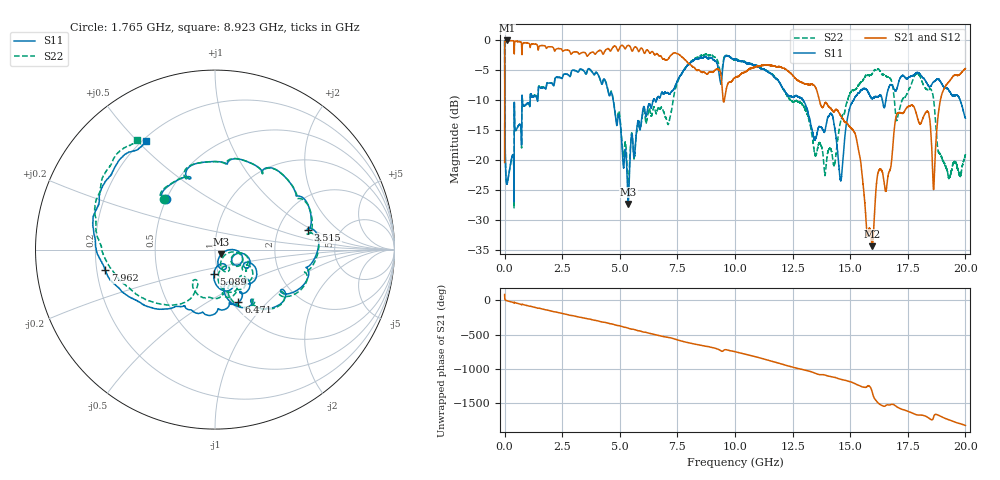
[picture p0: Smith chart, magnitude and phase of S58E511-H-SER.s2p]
!{S58E511}
!Johanson Technology Inc.
!www.johansontechnology.com
!Test Board Conditions:
!Substrate Type  RO4350B
!Substrate Thickness  60 mil
!Substrate Dk  3.66
!TL Type: GCPW
!TL Trace Width  115 mil
!TL Gap  52 mil
!Electrode orientation  Horizontal
!DUT TOPOLOGY	SERIES
!Mounting Pad LxW  55x428 mil
! Created Wed Apr 14 11:55:38 2021
# mhz S ma R 50
! 2 Port Network Data from SP1.SP block
! freq  magS11  angS11  magS21  angS21  magS12  angS12  magS22  angS22
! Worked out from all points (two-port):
!   20001 points, 300 kHz to 20 GHz, reference 50 ohm
!   highest |S21| = -0.02 dB at 99.3 MHz (marker M1); lowest = -34.4 dB at 15.95 GHz (marker M2)
!   |S21| within 3 dB of the highest: 3.17 MHz to 6.845 GHz (6.841 GHz wide, 200 % of centre); 7.119 GHz to 7.771 GHz (651.1 MHz wide, 8.75 % of centre)
!   lowest |S11| = -27.4 dB at 5.367 GHz (marker M3), VSWR 1.09, Z = 53.4 - j2.86 ohm
!   |S11| at or under -10 dB: 9.442 MHz to 750.8 MHz (741.4 MHz wide, 195 % of centre); 4.715 GHz to 6.451 GHz (1.736 GHz wide, 31.1 % of centre); 12.96 GHz to 15.15 GHz (2.19 GHz wide, 15.6 % of centre)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
!   |S22| runs from -28.1 to -0.1 dB; largest |S21 - S12| = 0.01
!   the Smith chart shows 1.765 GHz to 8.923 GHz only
!   S11 on the Smith chart (normalised r, x): 1.765 GHz: 0.49, +0.33; 3.515 GHz: 2.93, +0.90; 5.089 GHz: 0.95, -0.26; 6.471 GHz: 1.06, -0.70; 7.962 GHz: 0.23, -0.09; 8.923 GHz: 0.22, +0.53
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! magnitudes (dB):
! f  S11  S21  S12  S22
! 300 kHz  -0.1  -20.4  -20.4  -0.1
! 99.3 MHz  -23.9  0.0  0.0  -23.9
! 1.765 GHz  -8.1  -1.0  -1.0  -8.0
! 3.334 GHz  -4.8  -2.1  -2.1  -4.8
! 3.515 GHz  -5.5  -2.1  -2.1  -5.6
! 5.089 GHz  -17.3  -0.8  -0.8  -16.7
! 5.367 GHz  -27.4  -0.8  -0.8  -24.3
! 6.471 GHz  -9.9  -2.2  -2.2  -11.2
! 6.667 GHz  -9.4  -2.4  -2.5  -11.3
! 7.962 GHz  -4.1  -3.8  -3.7  -4.0
! 8.923 GHz  -2.9  -5.3  -5.3  -2.5
! 10 GHz  -3.2  -6.3  -6.3  -3.2
! 13.33 GHz  -14.8  -7.3  -7.3  -15.7
! 14.19 GHz  -12.4  -11.5  -11.4  -18.6
! 14.59 GHz  -23.4  -12.6  -12.6  -13.5
! 15.04 GHz  -10.6  -14.7  -14.7  -8.5
! 15.95 GHz  -9.7  -34.4  -34.3  -5.6
! 16.67 GHz  -8.0  -22.2  -22.3  -6.2
! 17.63 GHz  -6.0  -10.9  -10.9  -7.7
! 18.63 GHz  -6.9  -24.5  -24.4  -10.3
! 19 GHz  -7.5  -8.7  -8.7  -20.0
! 20 GHz  -13.0  -4.7  -4.7  -19.0
